FUNCTION_BLOCK FB 16
TITLE = FactoryLink S7 Write
// KNOW_HOW_PROTECT
AUTHOR : LET
FAMILY : S7_H1
NAME   : S7_WRITE
VERSION: 1.0


VAR_INPUT
  ID      : WORD;                      // Connection number, taken from CO configuration
END_VAR

VAR_OUTPUT
  DONE    : BOOL;                      // True if no error from AG-SEND/RECV
  ERROR   : BOOL;                      // True if any error from AG-SEND/RECV
  STATUS  : WORD;                      // Error status from AG-RECV
END_VAR

VAR
  R_NDR   : BOOL;                      // Set when data retrieved
  R_ERROR : BOOL;                      // Set when there was an error by AG-RECV
  S_DONE  : BOOL;                      // Set when there AG-SEND completes a frame
  S_ERROR : BOOL;                      // Set when AG-SEND has an error
  S_ACT   : BOOL;                      // Trigger to send a new frame with AG-SEND
  Sending : BOOL;                      // Indicates that we are sending data
  Recv_Buf: STRUCT                     // Buffer to receive "Write" request
   Sys_ID   : WORD;                    // Must contain 'S5' chars
   Opcod1   : WORD;                    // Must contain the value b#(16,01)
   Opcod2   : WORD;                    // Must contain the value b#(03,03)
   Opcod3   : WORD;                    // Must contain the value b#(03,08)
   Org_ID   : BYTE;                    // Must contain the value 01 = DB request
   DB_No    : BYTE;                    // The target DB no. 1-255
   DW_No    : WORD;                    // The start offset = Start DW no. 0-2047
   Len      : WORD;                    // No of WORDs  1-112 are allowed for CP443/343
   End_blck : WORD;                    // End header info. must contain B#(255,02)
   Data     : ARRAY [0..8192] OF BYTE; // Real data from the H1 partner
  END_STRUCT ;
  Send_Buf: STRUCT                     // Send buffer for Write Reply's
   Sys_ID   : WORD := W#16#5335;       // Must contain 'S5' chars
   Opcod1   : WORD := W#16#1001;       // Must contain the value b#(16,01)
   Opcod2   : WORD := W#16#306;        // Must contain the value b#(03,04)
   Opcod3   : WORD := W#16#F03;        // Must contain the value b#(0f,03)
   Err_No   : BYTE;                    // Contains either 0 = OK or errorcode
   Emp_Blck : BYTE := B#16#FF;         // Always xff, Indicating empty block
   Emp_Len  : BYTE := B#16#7;          // Lenght of unused header info
   DispHead0: BYTE;                    // Not used byte part of header
   DispHead1: WORD;                    // Not used part of header
   DispHead2: WORD;                    // Not used part of header
  END_STRUCT;
  SFB_12    : SFB 12;                  // Local instance of SFB 12
  SFB_13    : SFB 13;                  // Local instance of SFB 13
END_VAR

VAR_TEMP
  Source_Ptr: ANY;                     // Pointer to the target Data in this PLC's DB
  Dest_Ptr  : ANY;                     // Pointer to the internal data buf with user data
  Recv_Ptr  : ANY;                     // Pointer to the recv area in this instance DB
  Send_Ptr  : ANY;                     // Pointer to send area in this instance DB
  EN_STATUS : BOOL;                    // Used only for EN, ENO operation
  Int_Var   : INT;                     // Temporary integer value
  R_LEN     : WORD;                    // No. of BYTES received
  Max_Adr   : DWORD;                   // Maximum allowed address
  DB_Offset : WORD;                    // DB Number offset for nr. > 255
  LADDR     : DWORD;                   // CP module logical Baseaddress, from System Configuration
  S5        : BOOL;                    // S5 Addressing mode, when true
  S_LEN     : WORD;                    // No. of BYTES to send
END_VAR

BEGIN
NETWORK
TITLE =

      SET;
      SAVE;
      =     #EN_STATUS;                // Save if any uses the EN, ENO status
      SET;                             // Make sure all info bits are zero
      R     #R_NDR;
      R     #S_DONE;
      R     #R_ERROR;
      R     #S_ERROR;
      R     #S_ACT;
      R     #S5;
      CLR;                             // Clear RLO bit
      L     0;                         // Reset error code
      T     #STATUS;
      L     2;                         // Remote id
      T     #LADDR;
//
// Prepare the needed ANY pointers, so most of the initialization are done now.
// Cannot use static area for ANY pointers, must use local variable and build them up
//
      L     W#16#1002;                 // S7 syntax ID and lentype = 10 hex
      T     LW     0;                  // Begin create ANY WORD Pointer type
      T     LW    10;                  // DestPtr
      T     LW    20;                  // Our local receivebuffer
      T     LW    30;                  // Our local send buffer
      L     8208;                      // Max len in bytes
      T     LW     2;                  // to Source_Ptr
      L     8192;                      // BYTE Lenght of receive buffer
      T     LW    22;                  // to Recv_ptr
      L     16;                        // BYTE Lenght of send_buffer, only header
      T     LW    32;                  // to Send_Ptr
      L     DINO;                      // our own instance DB no
      T     LW     4;                  // Source_Ptr is always in our own DB
      T     LW    24;                  // Recv_Ptr Too
      T     LW    34;                  // Same with Send_ptr
      L     W#16#8400;                 // DB area type pointer
      T     LW     6;                  // Are the same for all pointers
      T     LW    16;                  // set dest ptr
      T     LW    26;                  // set recv ptr
      T     LW    36;                  // set send ptr
      L     8;                         // start offset for recv_buf
      SLW   3;                         // adjust to a bit pointer
      T     LW    28;                  // set for recv_ptr
      L     8218;                      // start offset send_ptr
      SLW   3;
      T     LW    38;                  // set for send_ptr
	L     8218;                      // start offset for send pointer
      SRW   13;                         // just keep the higher part
      T     LB    37;
//
// See If there is anything to receive from the partner (a write request)
//
      CALL  SFB 13,db113 (
            EN_R   := TRUE,
            ID     := #ID,             // Connection ID from CO config.
            R_ID   := #LADDR,          // Module base adr. from System Config.
            NDR    := #R_NDR,          // Set if data received
            ERROR  := #R_ERROR,        // Set if there was an error
            STATUS := #STATUS,         // Receive status information
            RD_1   := #Recv_Ptr,       // Our newly build ANY pointer to our own DB
            LEN    := #R_LEN);         // No of databytes received
      A     #Sending;                  // May not receive, while sending
      JC    SKIP;
//
// Anything received ??
//
      AN    #R_NDR;
      JC    NERR;                      // skip if not
      A     #R_ERROR;
      JC    NERR;
      L     0;                         // reset offset
      T     #DB_Offset;
      L     16;
      L     #R_LEN;                    // Received 16 bytes or less
      >I    ;
      JC    ERR1;                      // Did not get a header, need header and data
      L     'S7';                      // This must be the in first 2 bytes
      L     #Recv_Buf.Sys_ID;
      <>I   ;
      JC    ERR1;
      L     0;                         // Clear first part of header info for next frame
      T     #Recv_Buf.Sys_ID;
      L     W#16#1001;                 // must contain this value
      L     #Recv_Buf.Opcod1;
      <>I   ;
      JC    ERR1;
      L     W#16#303;                  // and this
      L     #Recv_Buf.Opcod2;
      <>I   ;
      JC    ERR1;
      L     W#16#308;                  // and this
      L     #Recv_Buf.Opcod3;
      <>I   ;
      JC    ERR1;
      L     W#16#FF02;                 // and this too
      L     #Recv_Buf.End_blck;
      <>I   ;
      JC    ERR1;
      L     1;
      L     #Recv_Buf.Org_ID;          // We expect only DB, FB IB and QB indentifier
      >I    ;
      JC    ERR2;                      // Send a header with error-info to our partner
      L     4;
      <=I   ;
      JC    EVAL;                      // Normal addressing parameters
      L     120;                        // Check for addressing above 255
      L     #Recv_Buf.Org_ID;
      >I    ;
      JC    ERR2;                      // Send a header with error-info to our partner
      L     134;
      >I    ;
      JC    ERR2;                      // Check for flagbytes above 255
      L     #Recv_Buf.Org_ID;
      L     119;
      -I    ;                          // Number of blocks
      L     256;                       // Block size of 256
      *I    ;                          // Offset
      T     #DB_Offset;                 // Activate offset
      L     1;
      T     #Recv_Buf.Org_ID;          // Adjust org id to normal value
//
// Evaluate received identifier
//
EVAL: L     1;
      L     #Recv_Buf.Org_ID;          // Evaluat DB indentifier
      <I    ;
      JC    I_FB;
      AN    #S5;                       // Check for word boundary
      JC    I_DB;
      L     #Recv_Buf.DW_No;           // Start address is to be doubled
      SLW   1;
      T     #Recv_Buf.DW_No;
      L     #Recv_Buf.Len;             // Length is to be doubled
      SLW   1;
      T     #Recv_Buf.Len;
I_DB: L     #Recv_Buf.DB_No;           // DB-number must be > 1
      L     DINO;                      // Our own Instance datablock no
      ==I   ;                          // May not be written to
      JC    ERR2;
      L     L#+65534;                  // Max. address
      T     #Max_Adr;
      JU    ADDR;                      // Go check address
I_FB: L     0;                         // Not a DB so set DBNR to zero
      T     #Recv_Buf.DB_No;
      L     2;
      L     #Recv_Buf.Org_ID;          // Evaluat FB indentifier
      <I    ;
      JC    I_IB;
      L     W#16#8300;                 // FB area type pointer
      T     LW    16;
      L     L#+2047;                   // Max. address
      T     #Max_Adr;
      JU    ADDR;                      // Go check address
I_IB: L     3;
      L     #Recv_Buf.Org_ID;          // Evaluat FB indentifier
      <I    ;
      JC    I_QB;
      L     W#16#8100;                 // IB area type pointer
      T     LW    16;
      L     L#+8191;                   // Max. address
      T     #Max_Adr;
      JU    ADDR;                      // Go check address
I_QB: L     W#16#8200;                 // QB area type pointer
      T     LW    16;
      L     L#+8191;                   // Max. address
      T     #Max_Adr;
ADDR: L     #Max_Adr;                  // Check begin address
      L     #Recv_Buf.DW_No;
      <D    ;
      JC    ERR2;
      L     0;
      L     #Recv_Buf.Len;             // Must be 1..112 datawords (224 bytes max)
      >=I   ;
      JC    ERR2;
      +     16;                        // Add the lenght of the H1 header
      L     #R_LEN;                    // Total no. of bytes received from partner
      <>I   ;                          // Something is wrong if they differ
      JC    ERR2;
      L     8208;
      >I    ;
      JC    ERR2;
//
// Copy from local DB to our own instance DB's Sendbuffer
//
      L     24;                        // Start offset for Source_ptr = Data[0]
      SLW   3;
      T     LW     8;                  // Now set for Source_Ptr
      L     #Recv_Buf.Len;             // No. of words
      T     LW    12;                  // Max words to pointer
      L     #Recv_Buf.DB_No;           // Get target DB
      L     #DB_Offset;                 // Add DB offset
      +I    ;
      T     LW    14;                  // To source ptr
      L     #Recv_Buf.DW_No;           // Get target DW
      SLD   3;                         // Adjust for Words and Pointer
      T     LW    18;                  // To source ptr
      SRD   16;                        // Get first three bits
      L     7;
      AW    ;                          // Remove not used bits
      T     LB    17;

      CALL  SFC   20 (
            SRCBLK  := #Source_Ptr,
            RET_VAL := #Int_Var,
            DSTBLK  := #Dest_Ptr);

      L     #Int_Var;                  // Get result from the block move
      L     0;                         // Should be Zero if OK.
      T     #Send_Buf.Err_No;          // In case there is no error
      ==I   ;
      JC    CONT;                      // Ok Continue if every thing is fine
      JU    ERR2;
ERR1: L     6;
      JU    CONT;
ERR2: L     3;                         // *** Errorcode. We use 3 only ***
CONT: T     #Send_Buf.Err_No;
//
// Create the H1 Fetch reply header information to make sure it is set up
//
      L     'S7';
      T     #Send_Buf.Sys_ID;
      L     W#16#1001;
      T     #Send_Buf.Opcod1;
      L     W#16#304;
      T     #Send_Buf.Opcod2;
      L     W#16#F03;
      T     #Send_Buf.Opcod3;
      L     B#16#FF;
      T     #Send_Buf.Emp_Blck;
      L     B#16#7;
      T     #Send_Buf.Emp_Len;
      SET   ;
      =     #S_ACT;
      S     #Sending;
//
// Send the requested data to the active partner
//
SKIP: NOP   0;
      L     2;                         //Remote id
      T     #LADDR;
      L     16;                        //Length of acknowledge telegram
      T     #S_LEN;
      CALL  SFB 12,db112 (
            REQ    := #S_ACT,
            R      := FALSE,
            ID     := #ID,
            R_ID   := #LADDR,
            DONE   := #S_DONE,
            ERROR  := #S_ERROR,
            STATUS := #STATUS,
            SD_1   := #Send_Ptr,
            LEN    := #S_LEN);
//
// The send function returns with a unknown error kode H7000
// after completing a sendjob or when not doing anything
// For now we just shortcircuit this problem but it must be solved by Siemens
//
      L     #STATUS;                   // Get send status
      L     W#16#7000;                 // Not Know error status
      <>I   ;                          // skip if not unknown status
      JC    NERR;
      L     W#16#8181;                 // force default status
      T     #STATUS;                   // Into the status info
      A     #S_ERROR;                  // and clear the error indikation
      R     #S_ERROR;
      R     #Sending;
//
// Final work before exit from this function
//
NERR: L     W#16#0;
      O     #S_DONE;
      O     #R_ERROR;
      JC    NO_R;
      JU    NO_S;
NO_R: AN    #S_ERROR;
      JC    NO_S;
NO_S: A     #S_DONE;
      =     #DONE;                     // Mark done flag
      A     #S_DONE;                   // Enable Reception after job completed or
      O     #S_ERROR;                  // there was an error
      R     #Sending;
      O     #R_ERROR;                  // error indication on either AG-RECV or AG-SEND
      O     #S_ERROR;
      AN    #S_DONE;
      =     #ERROR;                    // are send out
      A     #S_DONE;
      R     #S_DONE;
      A     #S_ERROR;
      R     #S_ERROR;
      CLR   ;                          // restore the EN status to ENO
      A     #EN_STATUS;
      SAVE  ;
END_FUNCTION_BLOCK
